TYPE ConfigHeater :
STRUCT
	HeaterTolerance_Enable:BOOL;
	HeaterAlarmRange:SVINT;
	HeaterAlarmTime:SVINT;
	HeaterWarningRange:SVINT;
	HeaterWarningTime:SVINT;
(*	
	TempOffsetPoint1:SVINT;
		OffsetValue1:SVLREAL;
		
	TempOffsetPoint2:SVINT;
		OffsetValue2:SVLREAL;
		
	TempOffsetPoint3:SVINT;
		OffsetValue3:SVLREAL;
		
	TempOffsetPoint4:SVINT;
		OffsetValue4:SVLREAL;
		
	TempOffsetPoint5:SVINT;
		OffsetValue5:SVLREAL;
		
	TempOffsetPoint6:SVINT;
		OffsetValue6:SVLREAL;
		
	TempOffsetPoint7:SVINT;
		OffsetValue7:SVLREAL;
		
	TempOffsetPoint8:SVINT;
		OffsetValue8:SVLREAL;
		
	TempOffsetPoint9:SVINT;
		OffsetValue9:SVLREAL;
		
	TempOffsetPoint10:SVINT;
		OffsetValue10:SVLREAL;
		*)
END_STRUCT
END_TYPE
